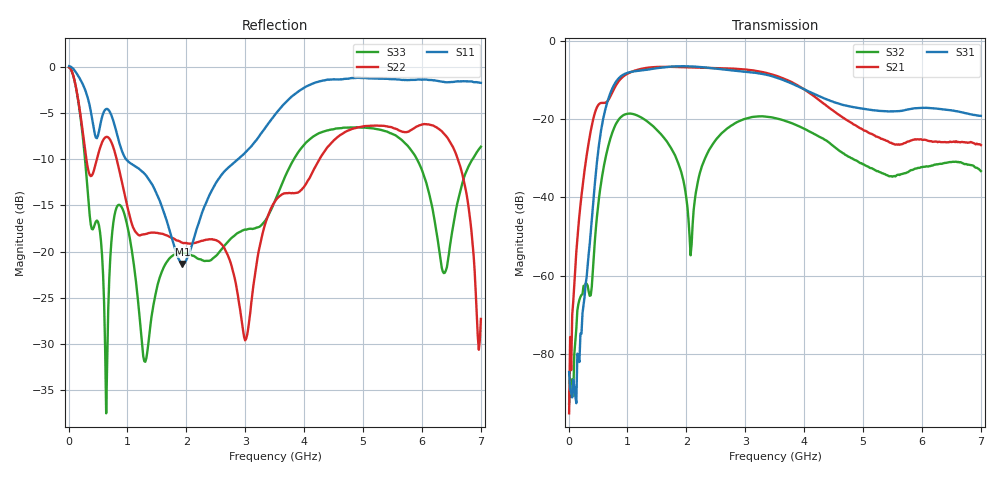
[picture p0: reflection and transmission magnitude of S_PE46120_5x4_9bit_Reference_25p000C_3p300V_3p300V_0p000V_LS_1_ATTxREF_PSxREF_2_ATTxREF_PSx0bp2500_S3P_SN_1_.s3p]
! Device ID: PE46120_5x4_9bit_Reference
! Device ID: PE46120_5x4_9bit_Reference
! File Path: z:\PE46120_5x4_9bit_Reference\MPAC_Yi\new_12port\25p000C\3p300\LS_1_ATTxREF_PSxREF_2_ATTxREF_PSx0bp2500\PE46120_5x4_9bit_Reference_25p000C_3p300V_3p300V_0p000V_LS_1_ATTxREF_PSxREF_2_ATTxREF_PSx0bp2500_S3P_SN_1_.s3p
! Serial: 1
! Lot:
! Temp: 25.000C
! VDD: 3.300
! VSS: 0.000
! Control_Hi: 3.300
! Control_Lo: 0.000
! Logic State: LS_1_ATTxREF_PSxREF_2_ATTxREF_PSx0bp2500
! Port 1: RFin
! Port 2: RFout1
! Port 3: RFout2
! ThroughPath:1-3
! IDD: -0.0005466189
! ISS: 0
! Comment:
#  Hz  S  RI  R  50
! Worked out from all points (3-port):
!   401 points, 10 MHz to 7 GHz, reference 50 ohm
!   strongest paths, dB at 10 MHz, 1.758 GHz, 3.505 GHz, 5.253 GHz, 7 GHz:
!     S31: -84.6, -6.6, -9.3, -17.8, -19.2
!     S21: -95.2, -6.7, -8.8, -24.6, -26.6
!     S32: -92.7, -27.9, -19.7, -33.3, -33.3
!   lowest |S11| = -21.3 dB at 1.932 GHz (marker M1), VSWR 1.19, Z = 59 + j2.69 ohm
!   |S11| at or under -10 dB: 976.6 MHz to 2.878 GHz (1.901 GHz wide, 98.6 % of centre)
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1e7  1.001 -0.115  0.0001 -5.41e-05  -6.24e-05 -0.000105
     1.68e-05 4.52e-06  0.9873 -0.0963  -3.08e-05 -3.14e-05
     -4.1e-05 -4.2e-05  2.31e-05 -2.26e-06  0.9873 -0.0965
2.37175e8  -0.4728 -0.6582  -0.0126 -0.00494  0.000145 0.000236
           -0.0126 -0.00507  -0.2897 -0.3522  -0.000338 0.000624
           0.000165 0.000288  -0.000224 0.000536  -0.2707 -0.3388
4.6435e8  -0.4072 -0.072  -0.0571 0.1163  0.0204 -0.00244
          -0.0572 0.118  0.1372 0.2688  -0.00217 0.00335
          0.0206 -0.00265  -0.00228 0.00332  0.1446 0.0169
9.36175e8  -0.2516 0.2177  0.3452 -0.0533  -0.0412 0.3659
           0.349 -0.0545  -0.0402 -0.2114  -0.0429 0.1031
           -0.0405 0.3695  -0.0428 0.1042  0.0577 -0.1539
1.93225e9  0.0827 0.0226  -0.4042 0.2101  -0.2971 -0.3631
           -0.4086 0.213  -0.1012 0.0476  -0.00129 0.0182
           -0.301 -0.3664  -0.00102 0.0185  0.0119 -0.0979
2.07205e9  0.0895 -0.0509  -0.2899 0.3474  -0.4174 -0.2093
           -0.2926 0.3519  -0.0656 0.0889  0.00166 -0.000352
           -0.4223 -0.2105  0.00177 -0.000412  -0.0327 -0.0905
2.473975e9  -0.00433 -0.2266  0.1804 0.4067  -0.3476 0.2667
            0.183 0.4112  0.0807 0.0836  -0.0423 0.0274
            -0.3507 0.2705  -0.0428 0.0278  -0.0828 0.0427
3.505e9  -0.3995 -0.3791  -0.0874 -0.3464  0.3375 -0.0417
         -0.0889 -0.3505  0.0587 0.1773  -0.0174 -0.1008
         0.3412 -0.043  -0.018 -0.1016  -0.0358 -0.1854
6.248575e9  -0.38 0.7496  0.0377 -0.0337  0.0319 0.131
            0.0387 -0.0342  0.4605 -0.0951  -0.0256 0.0035
            0.0329 0.1322  -0.0262 0.00361  -0.0283 -0.1228
7e9  -0.0975 0.8127  -0.0258 -0.0381  0.1076 0.00831
     -0.0266 -0.0382  -0.0353 0.025  0.0209 0.000486
     0.1097 0.00788  0.0217 0.00053  0.1143 0.3515
